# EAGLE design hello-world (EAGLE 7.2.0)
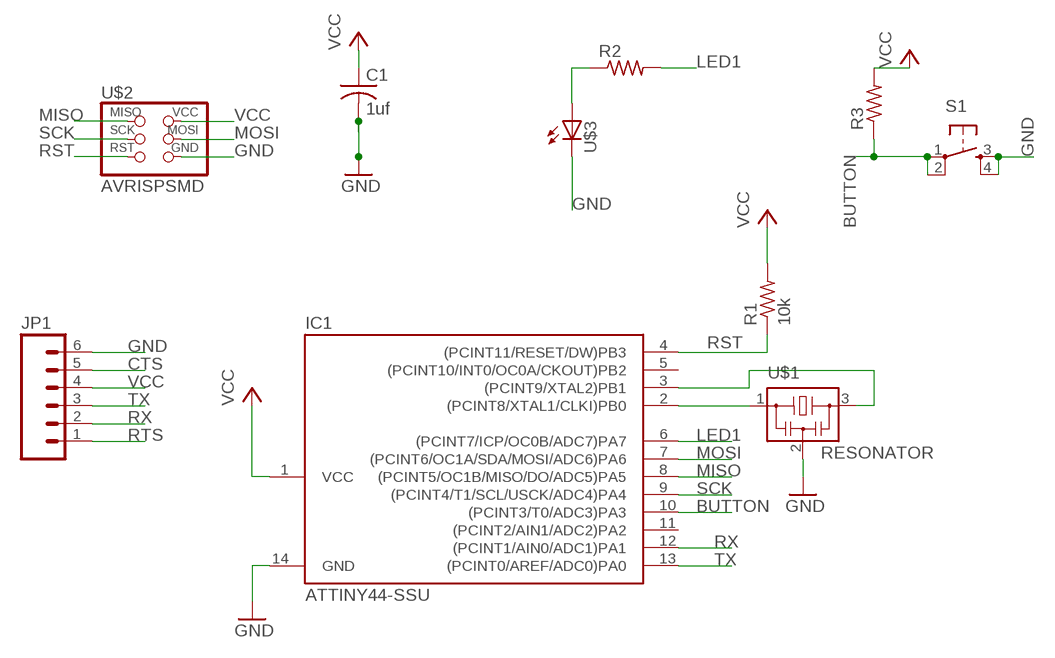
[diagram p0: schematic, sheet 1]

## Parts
C1  1uf  C-USC1206  [C1206]
IC1  ATTINY44-SSU  [SOIC14]
JP1  M06SMD  [1X06-SMD]
R1  10k  R-US_R1206  [R1206]
R2  RESISTOR1206  [1206]
R3  RESISTOR1206  [1206]
S1  6MM_SWITCH6MM_SWITCH  [6MM_SWITCH]
U$1  RESONATOR  [EFOBM]
U$2  AVRISPSMD  [2X03SMD]
U$3  LED1206  [1206]

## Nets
BUTTON: IC1.10((PCINT3/T0/ADC3)PA3) R3.1 S1.1(P) S1.2(P1)
CTS: JP1.5
GND: C1.2 IC1.14(GND) JP1.6 S1.3(S) S1.4(S1) U$1.2 U$2.6(GND) U$3.2(C)
LED1: IC1.6((PCINT7/ICP/OC0B/ADC7)PA7) R2.2
MISO: IC1.8((PCINT5/OC1B/MISO/DO/ADC5)PA5) U$2.1(MISO)
MOSI: IC1.7((PCINT6/OC1A/SDA/MOSI/ADC6)PA6) U$2.4(MOSI)
N$1: IC1.2((PCINT8/XTAL1/CLKI)PB0) U$1.1
N$2: IC1.3((PCINT9/XTAL2)PB1) U$1.3
N$3: R2.1 U$3.1(A)
RST: IC1.4((PCINT11/RESET/DW)PB3) R1.1 U$2.5(RST)
RTS: JP1.1
RX: IC1.12((PCINT1/AIN0/ADC1)PA1) JP1.2
SCK: IC1.9((PCINT4/T1/SCL/USCK/ADC4)PA4) U$2.3(SCK)
TX: IC1.13((PCINT0/AREF/ADC0)PA0) JP1.3
VCC: C1.1 IC1.1(VCC) JP1.4 R1.2 R3.2 U$2.2(VCC)
Unconnected: IC1.5((PCINT10/INT0/OC0A/CKOUT)PB2) IC1.11((PCINT2/AIN1/ADC2)PA2)

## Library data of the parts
C1 = rcl:C-US: CAPACITOR, American symbol
IC1 = fab:ATTINY44
JP1 = SparkFun:M06: Header 6 Standard 6-pin 0.1" header. Use with straight break away headers (SKU : PRT-00116), right angle break away headers (PRT-00553), swiss pins (PRT-00743), machine pins (PRT-00117), and female headers (PRT-00115). Molex polarized connector foot print use with SKU : PRT-08094 with associated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
R1 = resistor:R-US_: RESISTOR, American symbol
R2 R3 = 01_FAB_Hello:RESISTOR
S1 = fab:6MM_SWITCH: OMRON SWITCH
U$1 = fab:RESONATOR
U$2 = fab:AVRISP
U$3 = 01_FAB_Hello:LED

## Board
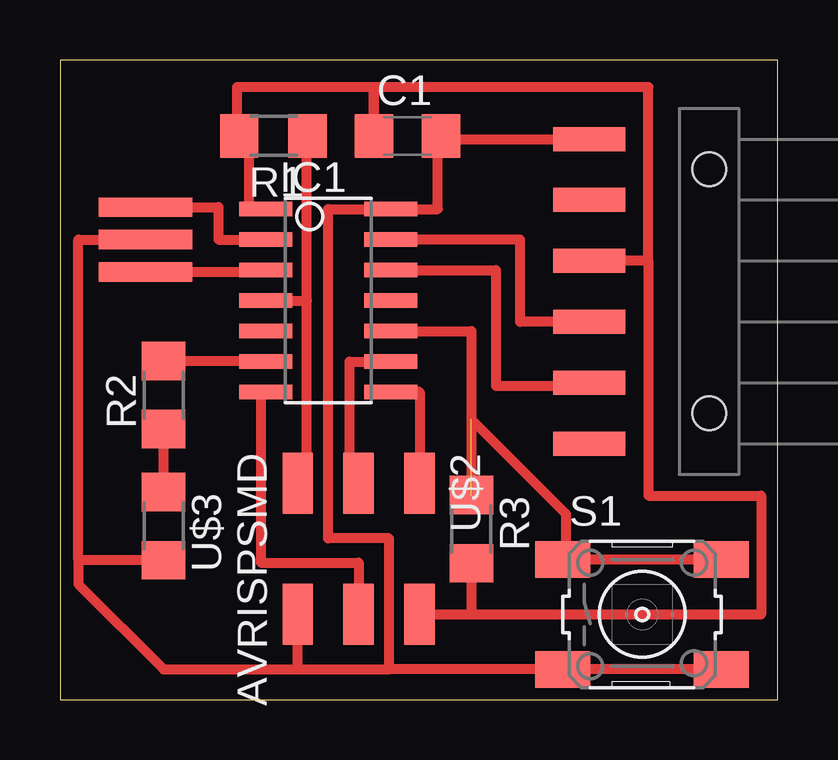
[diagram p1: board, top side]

Size 29.9 x 26.66 mm. Coordinates in mm from the lower left corner, seen from the top.
Outline: 0,0 29.9,0 29.9,26.66 0,26.66 0,0
Copper layers 1: Top 0.035mm
Design rules "ERP-1sided-10mil-16mill": minimum track width 10mil, minimum drill 24mil, track to track 16mil, track to pad 16mil, pad to pad 16mil, via to via 16mil, smd to smd 0mil, copper to edge 16mil, drill to drill 36mil, minimum pad ring 10mil, minimum via ring 8mil, stop-mask expansion 4mil, vias tented up to drill 0mil, thermal gap 10mil

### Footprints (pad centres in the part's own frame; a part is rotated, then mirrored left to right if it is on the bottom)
C1206 = smd 1.6 x 1.8: 1 -1.4,0; 2 1.4,0
SOIC14 = smd 0.61 x 2.21: 1 -3.81,-2.603; 2 -2.54,-2.603; 3 -1.27,-2.603; 4 0,-2.603; 5 1.27,-2.603; 6 2.54,-2.603; 7 3.81,-2.603; 8 3.81,2.603; 9 2.54,2.603; 10 1.27,2.603; 11 0,2.603; 12 -1.27,2.603; 13 -2.54,2.603; 14 -3.81,2.603
1X06-SMD = smd 1 x 3: 1 -6.35,5; 2 -3.81,5; 3 -1.27,5; 4 1.27,5; 5 3.81,5; 6 6.35,5 | hole 1.4: -5.08,0; 5.08,0
R1206 = smd 1.6 x 1.803: 1 -1.422,0; 2 1.422,0
1206 = smd 1.6 x 1.803: 1 -1.422,0; 2 1.422,0
6MM_SWITCH = smd 2.286 x 1.524: 1 -3.302,2.286; 2 3.302,2.286; 3 -3.302,-2.286; 4 3.302,-2.286
EFOBM = smd 0.8 x 3.9: 1 -1.35,0; 2 0,0; 3 1.35,0
2X03SMD = smd 2.54 x 1.27: 1 -2.54,2.54; 2 2.92,2.54; 3 -2.54,0; 4 2.92,0; 5 -2.54,-2.54; 6 2.92,-2.54

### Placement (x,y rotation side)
C1  14.48,23.5 0 top
IC1  11.18,16.64 270 top
JP1  27.05,17.02 90 top
R1  8.89,23.5 180 top
R2  4.32,12.7 90 top
R3  17.14,7.11 270 top
S1  24.26,3.56 0 top
U$1  3.56,19.18 270 top
U$2  12.45,6.48 270 top
U$3  4.32,7.24 270 top

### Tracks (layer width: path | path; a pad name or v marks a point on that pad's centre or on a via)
BUTTON  (2 unrouted)
  Top 0.406: S1.2 S1.1 21.08,5.97 21.08,7.75 17.14,11.68 | IC1.10 17.14,15.37 17.14,8.76
GND
  Top 0.406: 13.72,1.27 13.72,6.73 11.18,6.73 11.18,20.45 IC1.14 15.75,20.45 15.75,23.5 C1.2 15.88,23.37 JP1.6 | 9.91,1.27 13.72,1.27 | U$1.2 0.76,19.18 0.76,5.82 | U$2.6 9.91,1.27 | 13.72,1.27 S1.3 S1.4 | U$3.2 0.76,5.82 | 0.76,5.82 0.76,4.83 4.32,1.27 9.91,1.27
LED1
  Top 0.406: R2.2 8.57,14.12 IC1.6
MISO
  Top 0.406: IC1.8 14.99,12.83 U$2.1
MOSI
  Top 0.406: IC1.7 8.38,12.83 8.38,5.71 12.45,5.71 U$2.4
N$1
  Top 0.406: U$1.1 6.6,20.53 6.6,19.18 IC1.2
N$2
  Top 0.406: U$1.3 8.57,17.83 IC1.3
N$3
  Top 0.406: U$3.1 R2.1
RST
  Top 0.406: R1.1 10.29,23.5 10.29,16.64 | IC1.4 10.29,16.64 | U$2.5 10.29,9.02 10.29,16.64
RX
  Top 0.406: IC1.12 18.16,17.91 18.16,13.08 22.05,13.08 JP1.2
SCK
  Top 0.406: U$2.3 12.06,9.02 12.06,14.1 IC1.9
TX
  Top 0.406: JP1.3 19.18,15.75 19.18,19.18 IC1.13
VCC
  Top 0.406: 24.51,18.29 JP1.4 | IC1.1 7.87,20.45 7.87,23.5 R1.2 7.37,23.5 7.37,25.53 13.08,25.53 C1.1 13.08,25.53 24.51,25.53 24.51,18.29 | 24.51,18.29 24.51,8.51 29.21,8.51 29.21,3.56 17.14,3.56 | U$2.2 15.11,3.56 17.14,3.56 | R3.2 17.14,3.56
